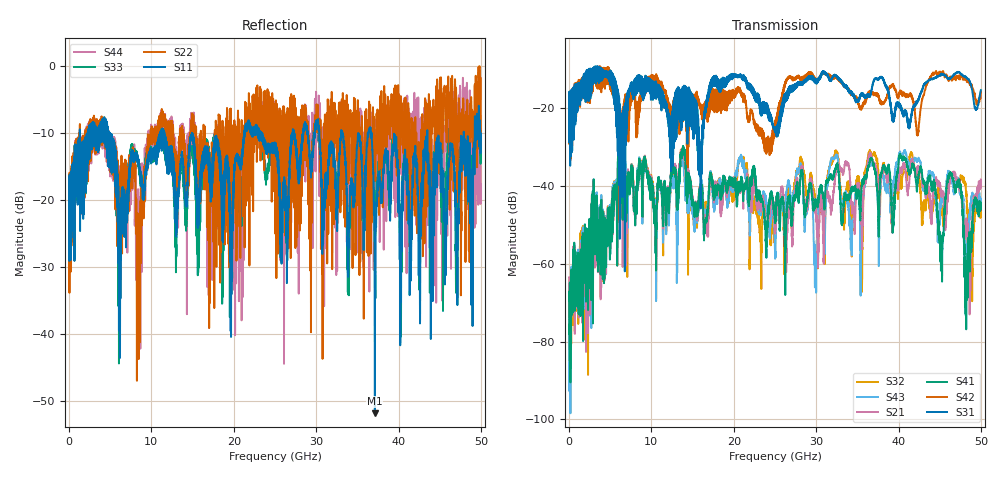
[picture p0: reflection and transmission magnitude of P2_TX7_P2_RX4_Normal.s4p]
!Keysight Technologies,N5225B,MY57041031,A.13.20.10
!Date: Friday, May 31, 2019 11:33:04
!Correction: S11(Full 4 Port(1,2,3,4))
!S12(Full 4 Port(1,2,3,4))
!S13(Full 4 Port(1,2,3,4))
!S14(Full 4 Port(1,2,3,4))
!S21(Full 4 Port(1,2,3,4))
!S22(Full 4 Port(1,2,3,4))
!S23(Full 4 Port(1,2,3,4))
!S24(Full 4 Port(1,2,3,4))
!S31(Full 4 Port(1,2,3,4))
!S32(Full 4 Port(1,2,3,4))
!S33(Full 4 Port(1,2,3,4))
!S34(Full 4 Port(1,2,3,4))
!S41(Full 4 Port(1,2,3,4))
!S42(Full 4 Port(1,2,3,4))
!S43(Full 4 Port(1,2,3,4))
!S44(Full 4 Port(1,2,3,4))
!S4P File: Measurements: <S11,S12,S13,S14>,
!<S21,S22,S23,S24>,
!<S31,S32,S33,S34>,
!<S41,S42,S43,S44>:
# Hz S  dB  R 50.0
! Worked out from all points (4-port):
!   5000 points, 10 MHz to 50 GHz, reference 50 ohm
!   strongest paths, dB at 10 MHz, 12.51 GHz, 25.01 GHz, 37.51 GHz, 50 GHz:
!     S31: -19.5, -22.3, -25.7, -12.7, -15.4
!     S42: -19.6, -28.0, -24.0, -16.8, -15.9
!     S41: -67.5, -37.0, -47.4, -45.9, -44.9
!     S21: -63.5, -36.6, -48.5, -39.6, -38.4
!     S43: -71.5, -39.6, -57.8, -45.2, -44.0
!     S32: -65.4, -39.3, -53.0, -35.5, -48.0
!   lowest |S11| = -51.8 dB at 37.13 GHz (marker M1), VSWR 1.01, Z = 50.2 + j0.125 ohm
!   |S11| at or under -10 dB: 4.911 GHz to 11.08 GHz (6.168 GHz wide, 77.1 % of centre); 11.57 GHz to 21.26 GHz (9.688 GHz wide, 59 % of centre); 36.73 GHz to 43.5 GHz (6.765 GHz wide, 16.9 % of centre)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
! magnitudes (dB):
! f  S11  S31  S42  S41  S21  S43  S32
! 10 MHz  -20.2  -19.5  -19.6  -67.5  -63.5  -71.5  -65.4
! 6.16 GHz  -26.7  -53.6  -32.8  -31.2  -32.4  -30.2  -31.2
! 28.06 GHz  -13.6  -14.0  -12.5  -38.6  -38.4  -34.5  -33.6
! 29.91 GHz  -9.1  -13.2  -12.7  -43.4  -46.1  -58.6  -45.1
! 37.13 GHz  -51.8  -12.5  -16.2  -35.6  -34.4  -35.4  -31.6
! 48.26 GHz  -13.7  -12.3  -12.6  -66.3  -51.3  -59.9  -43.0
! 50 GHz  -11.0  -15.4  -15.9  -44.9  -38.4  -44.0  -48.0
